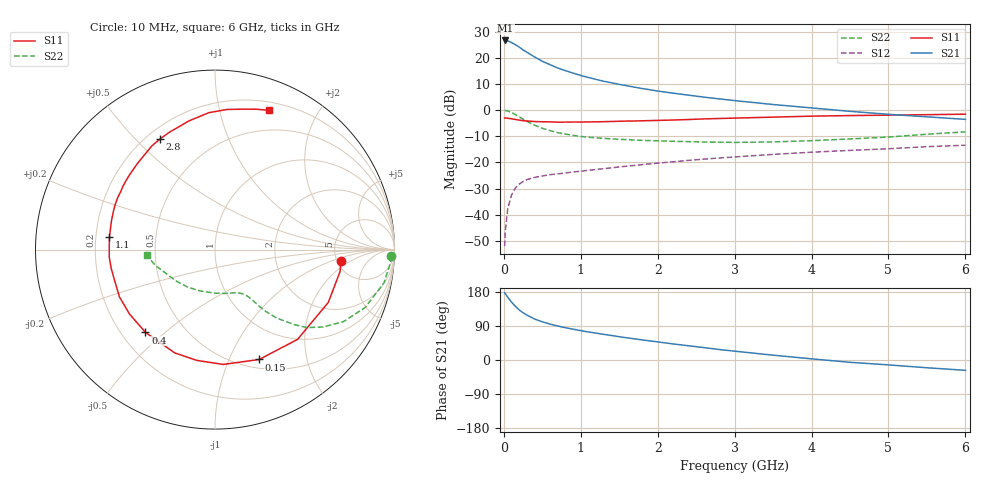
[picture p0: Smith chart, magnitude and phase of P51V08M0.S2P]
! SIEMENS Small Signal Semiconductors
! BFP183
! Si NPN RF Bipolar Junction Transistor in SOT143
! VCE = 1 V  IC = 8 mA
! Common Emitter S-Parameters:  March  1996
# GHz  S  MA  R  50
!  f  S11  S21  S12  S22
! GHz  MAG  ANG  MAG  ANG  MAG  ANG  MAG  ANG
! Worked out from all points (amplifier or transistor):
!   36 points, 10 MHz to 6 GHz, reference 50 ohm
!   highest |S21| = 26.6 dB at 20 MHz (marker M1)
!   |S21| within 3 dB of that: start of sweep to 221.2 MHz
!   unconditionally stable (mu >= 1): 1.163 GHz to end of sweep
!   at 250 MHz: K = 0.30, MSG = 25.2 dB, |S12| = -27.4 dB
!   at 1.4 GHz: K = 1.08, MAG = 14.5 dB, |S12| = -22.1 dB
!   at 6 GHz: K = 1.01, MAG = 4.2 dB, |S12| = -13.5 dB
!   S11 on the Smith chart (normalised r, x): 10 MHz: 5.45, -1.36; 150 MHz: 0.60, -1.30; 400 MHz: 0.30, -0.43; 1.1 GHz: 0.26, +0.06; 2.8 GHz: 0.25, +0.59; 6 GHz: 0.28, +1.42
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0.01  0.706 -5.1  21.28 177.3  0.0025 82.3  0.9838 -2.2
0.02  0.7072 -10.1  21.36 174.8  0.005 84.6  0.9795 -4.5
0.05  0.6965 -25.0  21.05 165.8  0.0129 79.4  0.9597 -11.1
0.1  0.6795 -47.4  19.42 152.9  0.0238 67.6  0.8965 -21.1
0.15  0.6599 -68.1  17.72 141.5  0.0323 59.6  0.8205 -29.3
0.2  0.6414 -85.9  15.91 132.1  0.0383 53.4  0.7405 -35.6
0.25  0.6256 -99.3  14.11 124.6  0.0429 48.2  0.6717 -40.3
0.3  0.6176 -111.3  12.68 118.4  0.0468 44.5  0.6082 -43.4
0.4  0.6025 -130.0  10.32 108.1  0.0515 40.0  0.513 -48.0
0.5  0.5964 -143.2  8.55 100.8  0.0549 37.1  0.448 -50.5
0.6  0.594 -153.7  7.361 94.8  0.0581 36.0  0.4037 -51.9
0.7  0.5853 -162.4  6.361 89.8  0.0602 35.5  0.3707 -52.8
0.9  0.5906 -175.9  5.08 81.4  0.0655 35.7  0.3276 -54.4
1.1  0.5922 173.0  4.187 73.9  0.0704 36.2  0.302 -56.4
1.5  0.6096 156.2  3.091 61.4  0.0817 37.2  0.2755 -61.2
1.8  0.6229 145.1  2.575 53.0  0.0905 37.6  0.2632 -66.4
2.2  0.6443 132.6  2.101 42.4  0.1024 36.8  0.2526 -74.6
2.8  0.6885 116.3  1.631 27.7  0.1212 34.3  0.2431 -90.1
3.5  0.7316 101.4  1.274 12.7  0.1419 30.4  0.2456 -111.0
4.5  0.7836 85.1  0.944 -6.1  0.1691 23.4  0.2799 -141.8
5.5  0.8152 73.6  0.741 -20.5  0.1995 16.8  0.3447 -165.3
6  0.8323 68.8  0.663 -27.2  0.2123 12.5  0.3825 -175.6
